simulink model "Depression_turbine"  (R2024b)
settings: Solver=ode15s  StartTime=0.0  StopTime=inf  RelTol=1e-3  EnableMultiTasking=on
libraries: fl_lib x7, nesl_utility x3

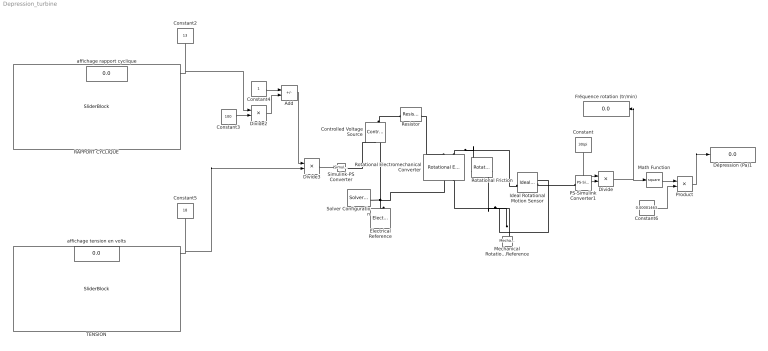
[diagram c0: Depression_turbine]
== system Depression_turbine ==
  Add : Sum  Inputs=+-
  Constant : Constant  Value=30/pi
  Constant2 : Constant  Value=13
  Constant3 : Constant  Value=100
  Constant4 : Constant
  Constant5 : Constant  Value=18
  Constant6 : Constant  Value=0.00001463
  Controlled Voltage Source : fl_lib/Electrical/Electrical Sources/Controlled Voltage Source
  Divide : Product  Inputs=**
  Divide2 : Product  Inputs=*/
  Divide3 : Product  Inputs=**
  Dépression (Pa)1 : Display
  Electrical Reference : fl_lib/Electrical/Electrical Elements/Electrical Reference
  Fréquence rotation (tr/min) : Display
  Ideal Rotational Motion Sensor : fl_lib/Mechanical/Mechanical Sensors/Ideal Rotational Motion Sensor  reference=foundation.enum.MeasurementReference.difference  acceleration_port=false  velocity_port=true  position_port=true  wrap_angle=false  offset=0 rad
  Math Function : Math  Operator=square
  Mechanical Rotational Reference : fl_lib/Mechanical/Rotational Elements/Mechanical Rotational Reference
  PS-Simulink Converter1 : nesl_utility/PS-Simulink Converter  PhysicalDomain=network_engine_domain  SubClassName=ps_output  LeftPortType=input  RightPortType=output  PseudoPeriodic=off  Frequencies=[]  VectorFormat=1-D array  Unit=rad/s  AffineConversion=off
  Product : Product
  RAPPORT CYCLIQUE : SliderBlock  Tag=rapport cyclique  LabelPosition=Hide  ScaleMin=10  ScaleMax=90  TickInterval=5
  Resistor : fl_lib/Electrical/Electrical Elements/Resistor  R=4.6 Ohm  i_specify=off  i_priority=High  i=0 A  i_nominal_specify=off  i_nominal_value=1  i_nominal_unit=A  v_specify=off  v_priority=High  v=0 V  v_nominal_specify=off  v_nominal_value=1  v_nominal_unit=V
  Rotational Electromechanical Converter : fl_lib/Electrical/Electrical Elements/Rotational Electromechanical Converter  K=0.01 V/(rad/s)  i_specify=off  i_priority=High  i=0 A  i_nominal_specify=off  i_nominal_value=1  i_nominal_unit=A  v_specify=off  v_priority=High  v=0 V  v_nominal_specify=off  v_nominal_value=1  v_nominal_unit=V  t_specify=off  t_priority=High  t=0 N*m  t_nominal_specify=off  t_nominal_value=1  t_nominal_unit=N*m  w_specify=off  w_priority=High  w=0 rad/s  w_nominal_specify=off  w_nominal_value=1  w_nominal_unit=rad/s
  Rotational Friction : fl_lib/Mechanical/Rotational Elements/Rotational Friction  brkwy_trq=0.00000001 N*m  brkwy_vel=0.1 rad/s  Col_trq=0.00000001 N*m  visc_coef=0.00001 N*m*s/rad  w_specify=off  w_priority=None  w=0 rad/s  w_nominal_specify=off  w_nominal_value=1  w_nominal_unit=rad/s  t_specify=off  t_priority=None  t=0 N*m  t_nominal_specify=off  t_nominal_value=1  t_nominal_unit=N*m
  Simulink-PS Converter : nesl_utility/Simulink-PS Converter  PhysicalDomain=network_engine_domain  SubClassName=ps_input  LeftPortType=input  RightPortType=output  PseudoPeriodic=off  Frequencies=[]  NoiseDistribution=none  NoiseParameters=[]  Unit=V  AffineConversion=off  FilteringAndDerivatives=provide  SimscapeFilterOrder=1  InputFilterTimeConstant=0.001  UdotUserProvided=0
  Solver Configuration : nesl_utility/Solver Configuration  PhysicalDomain=network_engine_domain  SubClassName=solver  LeftPortType=input  RightPortType=generic  Tones=[]  Harmonics=[]  SimulateNoise=off  Profile=off  UseLocalSampling=off  EnableSwitchedLinearOptims=on  FrequencyDomain=off  UseCCode=off  RelTol=0.001  AbsTol=1e-06  MinStep=1e-09  ToWorkspace=off  RevertToSquareIcSolve=off  NumHomotopyIterations=100  PhasorMode=off  PhasorModeNumHarmonics=1  ConsistencySolver=NEWTON_FTOL  IndexReductionMethod=DerivativeReplacement  DoDC=off  ResidualTolerance=1e-09  ConsistencyTolSource=GLOBAL  ConsistencyAbsTol=0.001  ConsistencyRelTol=0.001  ConsistencyTolFactor=0.001  UseLocalSolver=off  LocalSolverChoice=NE_BACKWARD_EULER_ADVANCER  ResolveIndetEquations=on  FunctionEvalNumThread=1  LocalSolverSampleTime=0.001  DoFixedCost=off  MaxNonlinIter=3  MaxModeIter=2  ComputeImpulses=off  ImpulseIterations=2  LinearAlgebra=Sparse  LinearAlgebraNumThread=0  EquationFormulation=NE_TIME_EF  DelaysMemoryBudget=1024  AutomaticFiltering=on  FilteringTimeConstant=0.001  PartitionStorageMethod=AS_NEEDED  PartitionMemoryBudget=1024  PartitionMethod=FAST  MultibodyUseLocalSolver=off  MultibodyLocalSolverChoice=ODE1  MultibodyLocalSolverSampleTime=0.001
  TENSION : SliderBlock  Tag=rapport cyclique  LabelPosition=Hide  ScaleMin=8  ScaleMax=26
  affichage rapport cyclique : Display
  affichage tension en volts : Display
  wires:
  Constant/1 -> Divide/1
  Divide/1 -> Math Function/1, Fréquence rotation (tr/min)/1
  Constant2/1 -> affichage rapport cyclique/1, Divide2/1
  Constant3/1 -> Divide2/2
  Constant4/1 -> Add/1
  Divide2/1 -> Add/2
  Add/1 -> Divide3/1
  Divide3/1 -> Simulink-PS Converter/1
  Constant5/1 -> affichage tension en volts/1, Divide3/2
  PS-Simulink Converter1/1 -> Divide/2
  Math Function/1 -> Product/1
  Constant6/1 -> Product/2
  Product/1 -> Dépression (Pa)1/1
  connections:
  Electrical Reference/LConn1 -- Solver Configuration/RConn1 -- Controlled Voltage Source/RConn2 -- Rotational Electromechanical Converter/RConn1
  Ideal Rotational Motion Sensor/RConn1 -- Mechanical Rotational Reference/LConn1 -- Rotational Friction/RConn1 -- Rotational Electromechanical Converter/RConn2
  Resistor/RConn1 -- Rotational Electromechanical Converter/LConn1
  Rotational Electromechanical Converter/LConn2 -- Ideal Rotational Motion Sensor/LConn1 -- Rotational Friction/LConn1
  Ideal Rotational Motion Sensor/RConn2 -- PS-Simulink Converter1/LConn1
  Simulink-PS Converter/RConn1 -- Controlled Voltage Source/RConn1
  Controlled Voltage Source/LConn1 -- Resistor/LConn1
